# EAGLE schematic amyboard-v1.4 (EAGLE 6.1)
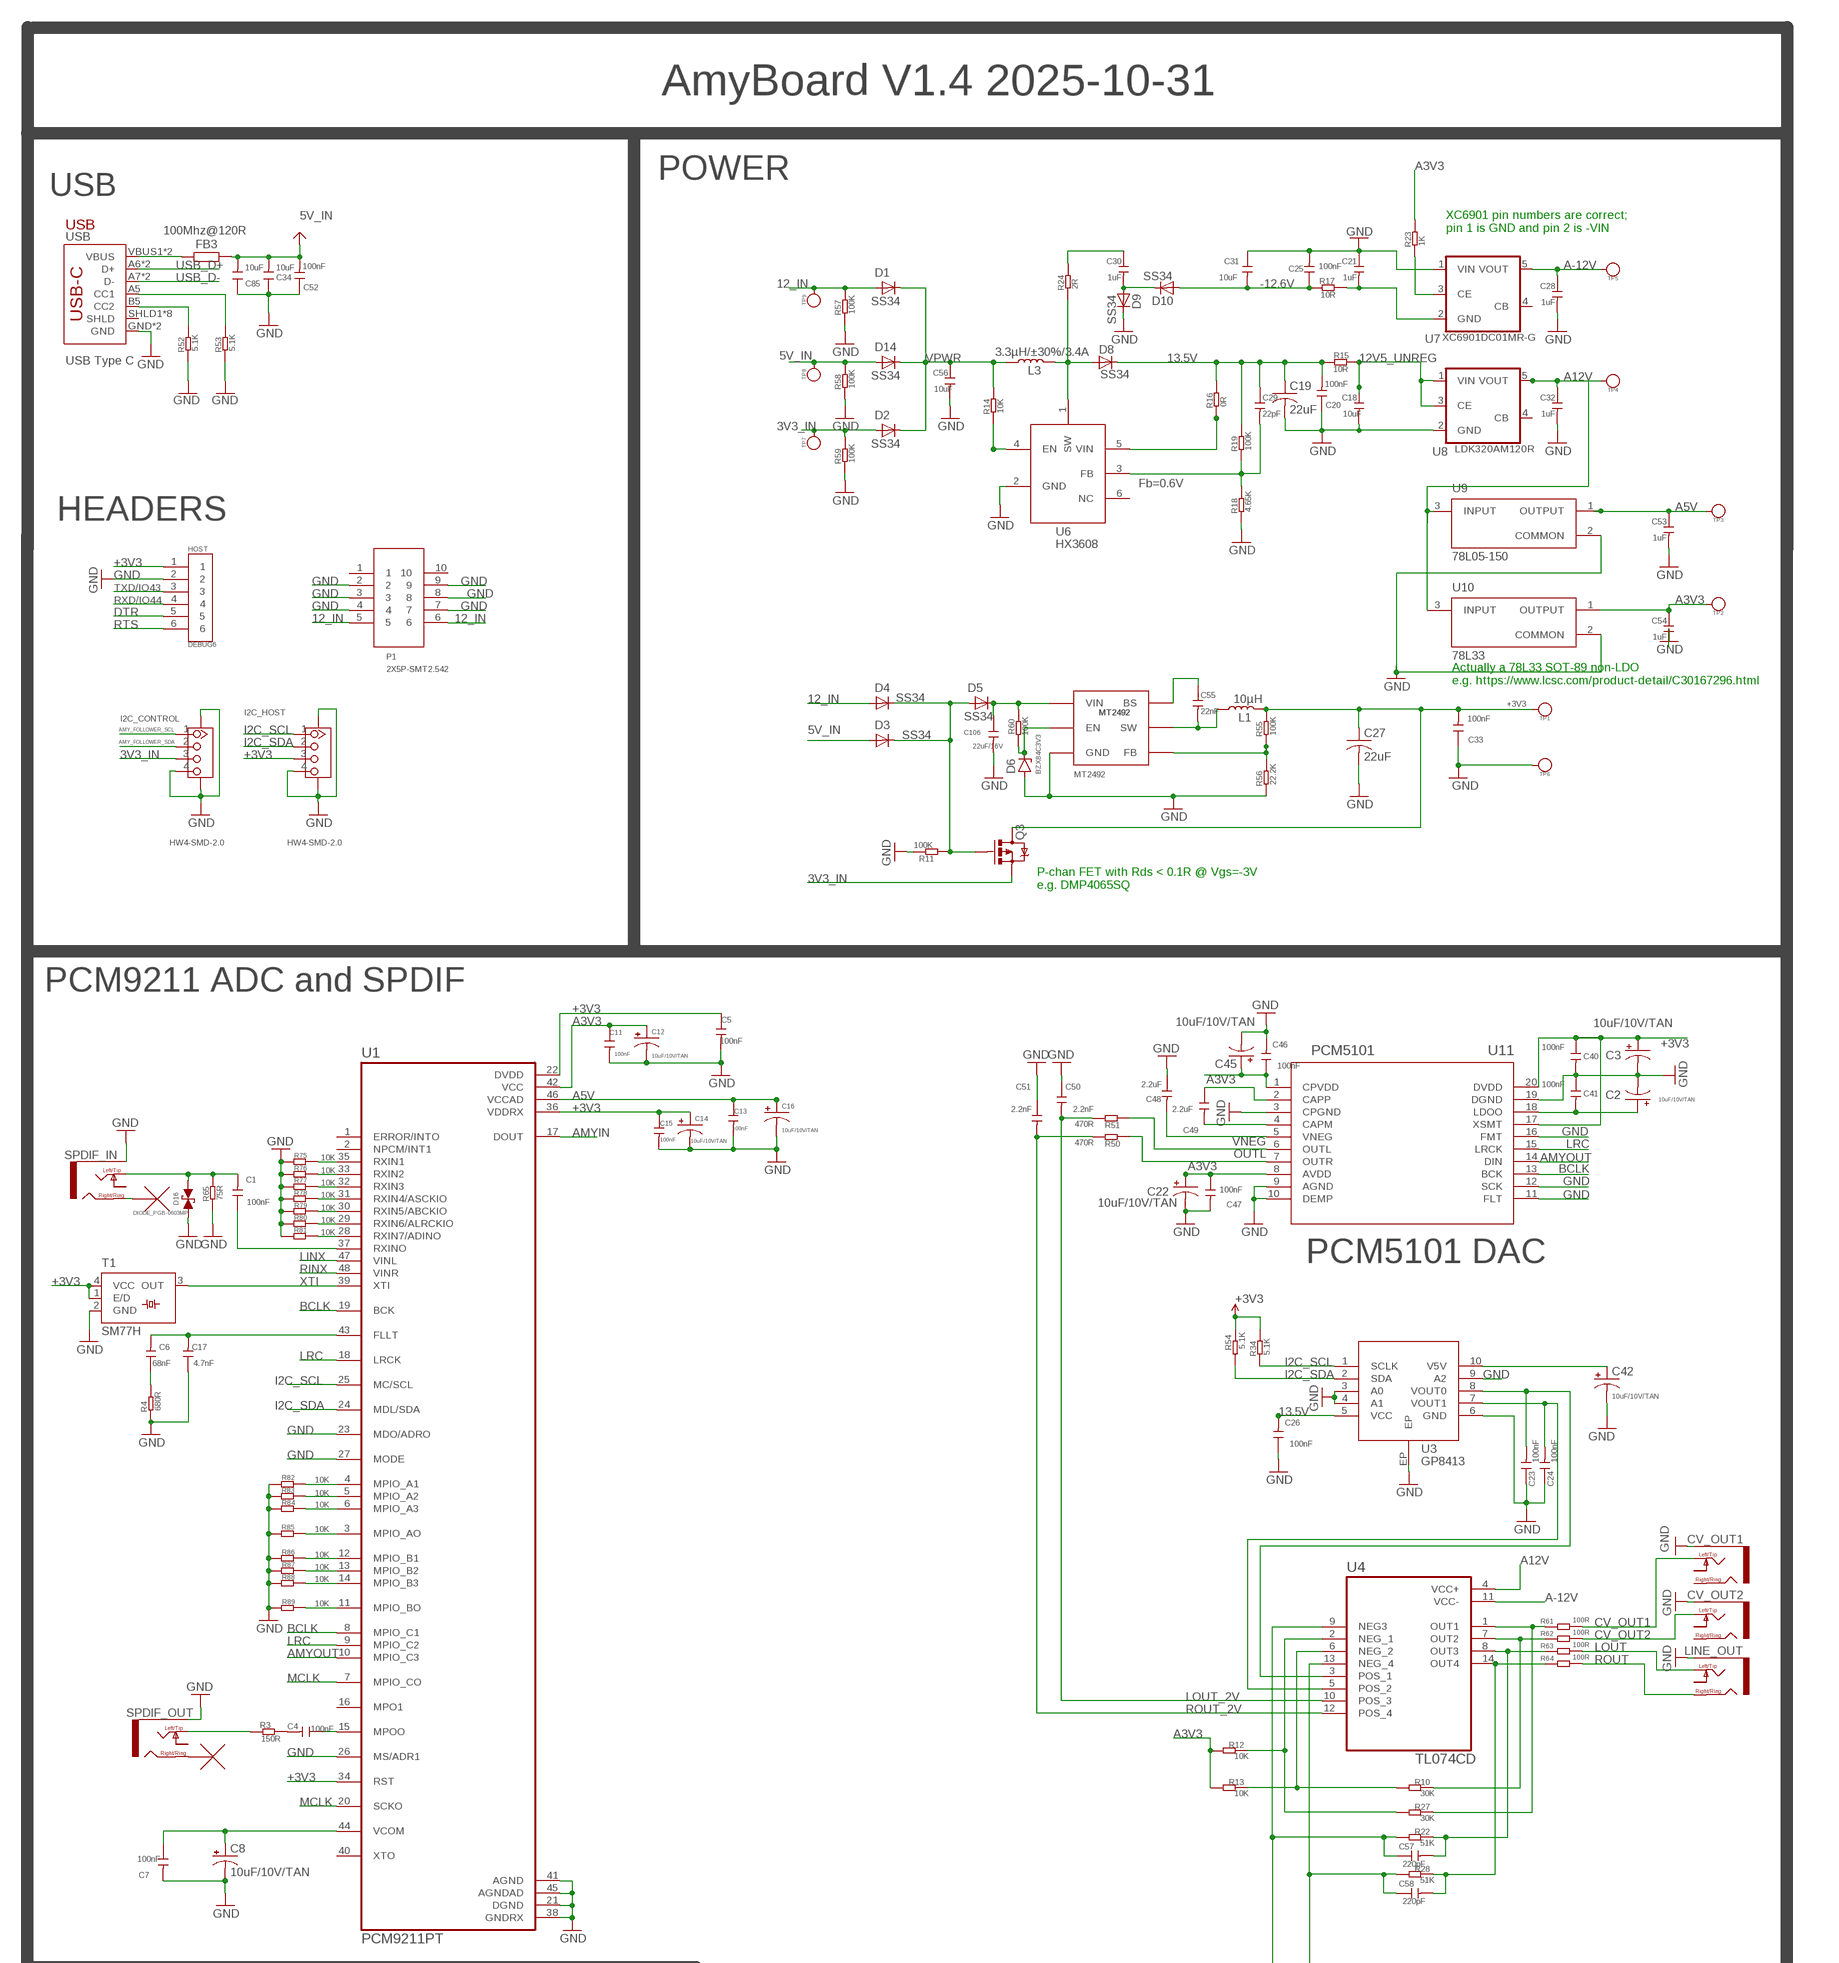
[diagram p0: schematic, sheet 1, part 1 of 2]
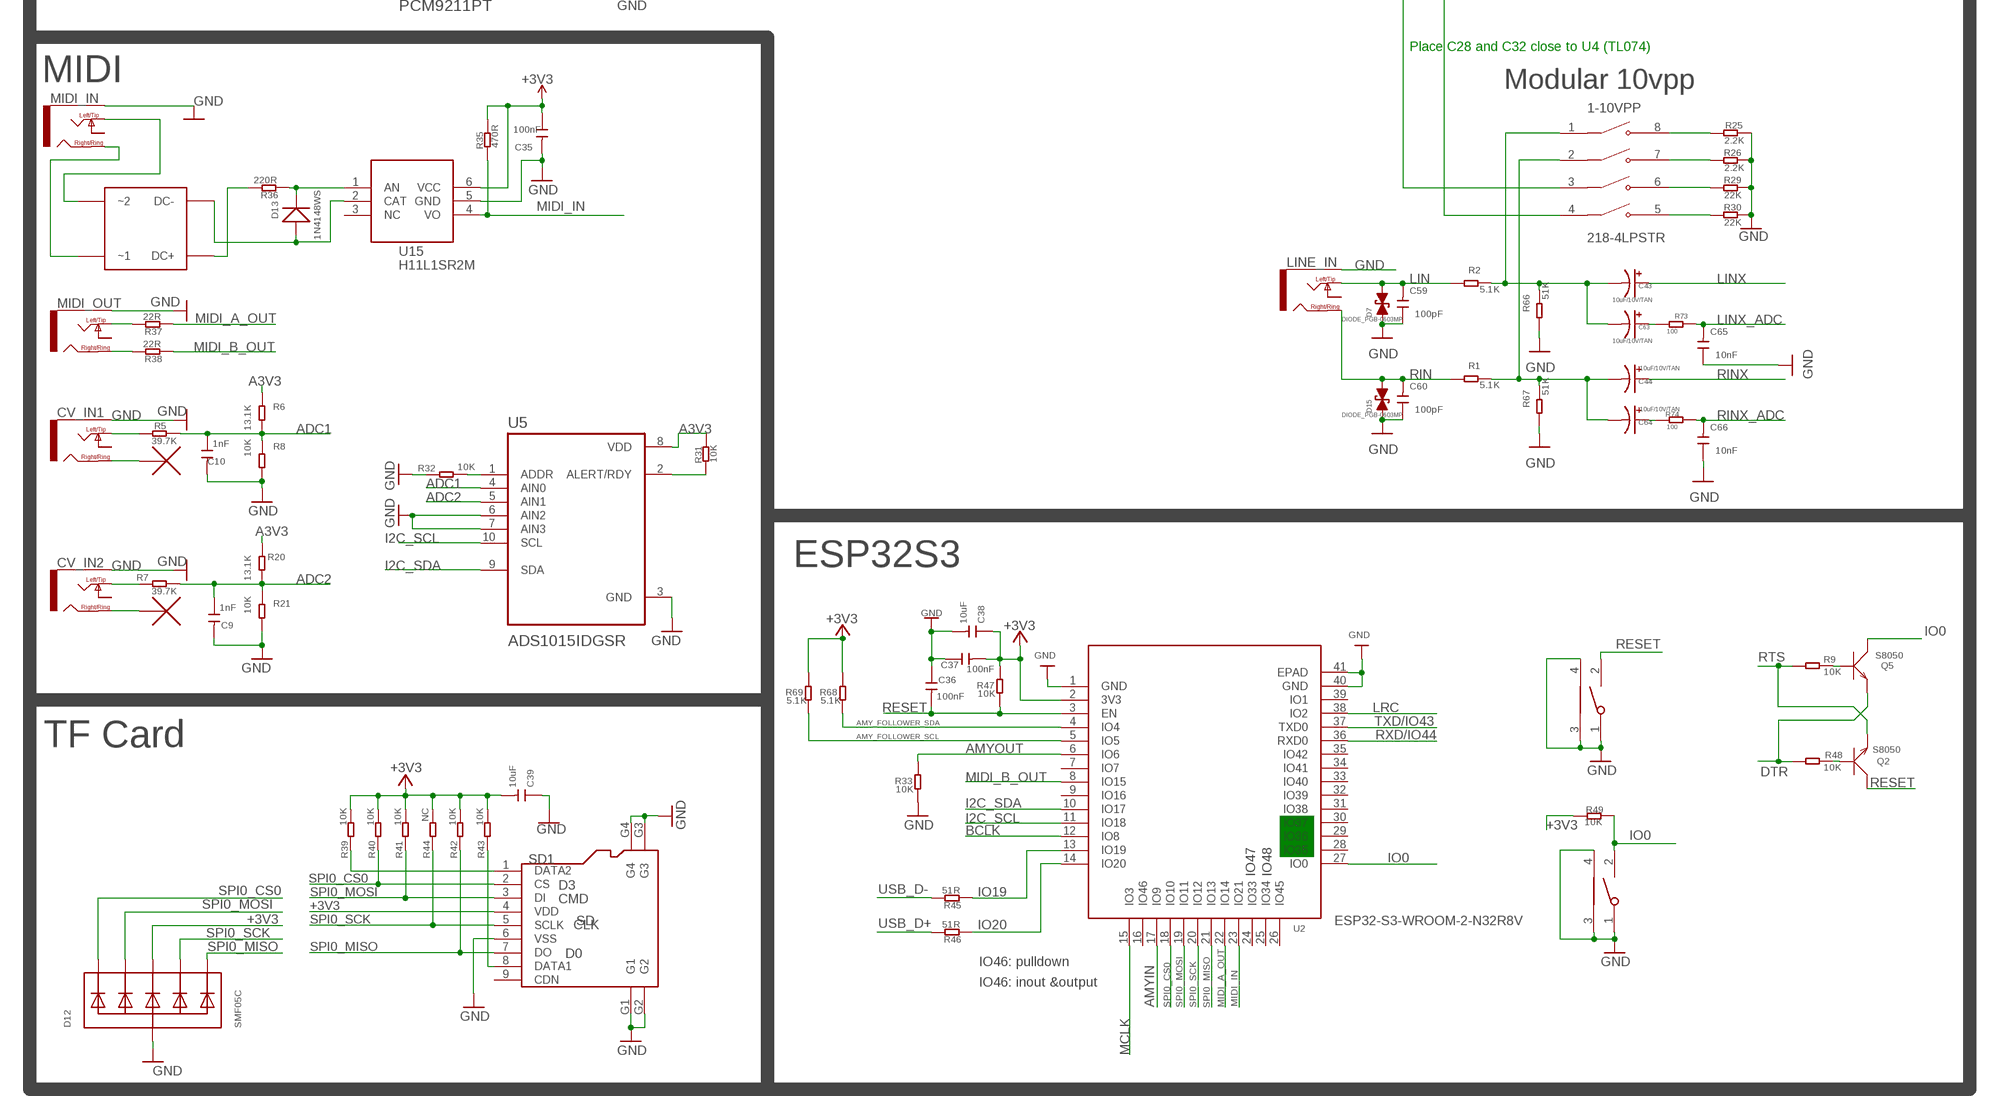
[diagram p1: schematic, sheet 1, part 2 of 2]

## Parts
1-10VPP  218-4LPSTR  [SW_218-4LPSTR]
BOOT  TS24CA  [2*4*3.5MM]
C1  100nF  DISCRETE_C-0402  [DISCRETE_C0402]
C2  10uF/10V/TAN  CPOL-USSMCZ  [SMC_Z]
C3  10uF/10V/TAN  CPOL-USSMCZ  [SMC_Z]
C4  100nF  DISCRETE_C-0402  [DISCRETE_C0402]
C5  100nF  DISCRETE_C-0402  [DISCRETE_C0402]
C6  68nF  DISCRETE_C-0402  [DISCRETE_C0402]
C7  100nF  DISCRETE_C-0402  [DISCRETE_C0402]
C8  10uF/10V/TAN  CPOL-USSMCZ  [SMC_Z]
C9  1nF  DISCRETE_C-0402  [DISCRETE_C0402]
C10  1nF  DISCRETE_C-0402  [DISCRETE_C0402]
C11  100nF  DISCRETE_C-0402  [DISCRETE_C0402]
C12  10uF/10V/TAN  CPOL-USSMCZ  [SMC_Z]
C13  100nF  DISCRETE_C-0402  [DISCRETE_C0402]
C14  10uF/10V/TAN  CPOL-USSMCZ  [SMC_Z]
C15  100nF  DISCRETE_C-0402  [DISCRETE_C0402]
C16  10uF/10V/TAN  CPOL-USSMCZ  [SMC_Z]
C17  4.7nF  DISCRETE_C-0402  [DISCRETE_C0402]
C18  10uF  CAP-0603  [C0603]
C19  22uF  C-USC1206  [C1206]
C20  100nF  DISCRETE_C-0402  [DISCRETE_C0402]
C21  1uF  CAP-0603  [C0603]
C22  10uF/10V/TAN  CPOL-USSMCZ  [SMC_Z]
C23  100nF  DISCRETE_C-0402  [DISCRETE_C0402]
C24  100nF  DISCRETE_C-0402  [DISCRETE_C0402]
C25  100nF  DISCRETE_C-0402  [DISCRETE_C0402]
C26  100nF  DISCRETE_C-0402  [DISCRETE_C0402]
C27  22uF  C-USC1206  [C1206]
C28  1uF  CAP-0603  [C0603]
C29  22pF  CAP-0603  [C0603]
C30  1uF  CAP-0603  [C0603]
C31  10uF  CAP-0603  [C0603]
C32  1uF  CAP-0603  [C0603]
C33  100nF  DISCRETE_C-0402  [DISCRETE_C0402]
C34  10uF  DISCRETE_C-0603  [DISCRETE_C0603]
C35  100nF  DISCRETE_C-0402  [DISCRETE_C0402]
C36  100nF  DISCRETE_C-0402  [DISCRETE_C0402]
C37  100nF  DISCRETE_C-0402  [DISCRETE_C0402]
C38  10uF  DISCRETE_C-0603  [DISCRETE_C0603]
C39  10uF  DISCRETE_C-0603  [DISCRETE_C0603]
C40  100nF  DISCRETE_C-0402  [DISCRETE_C0402]
C41  100nF  DISCRETE_C-0402  [DISCRETE_C0402]
C42  10uF/10V/TAN  CPOL-USSMCZ  [SMC_Z]
C43  10uF/10V/TAN  CPOL-USSMCZ  [SMC_Z]
C44  10uF/10V/TAN  CPOL-USSMCZ  [SMC_Z]
C45  10uF/10V/TAN  CPOL-USSMCZ  [SMC_Z]
C46  100nF  DISCRETE_C-0402  [DISCRETE_C0402]
C47  100nF  DISCRETE_C-0402  [DISCRETE_C0402]
C48  2.2uF  DISCRETE_C-0402  [DISCRETE_C0402]
C49  2.2uF  DISCRETE_C-0402  [DISCRETE_C0402]
C50  2.2nF  DISCRETE_C-0402  [DISCRETE_C0402]
C51  2.2nF  DISCRETE_C-0402  [DISCRETE_C0402]
C52  100nF  DISCRETE_C-0402  [DISCRETE_C0402]
C53  1uF  CAP-0603  [C0603]
C54  1uF  CAP-0603  [C0603]
C55  22nF  CAP-0603  [C0603]
C56  10uF  CAP-0603  [C0603]
C57  220pF  DISCRETE_C-0402  [DISCRETE_C0402]
C58  220pF  DISCRETE_C-0402  [DISCRETE_C0402]
C59  100pF  DISCRETE_C-0402  [DISCRETE_C0402]
C60  100pF  DISCRETE_C-0402  [DISCRETE_C0402]
C63  10uF/10V/TAN  CPOL-USSMCZ  [SMC_Z]
C64  10uF/10V/TAN  CPOL-USSMCZ  [SMC_Z]
C65  10nF  DISCRETE_C-0402  [DISCRETE_C0402]
C66  10nF  DISCRETE_C-0402  [DISCRETE_C0402]
C85  10uF  DISCRETE_C-0603  [DISCRETE_C0603]
C106  22uF/16V  C-0603  [0603]
CV_IN1  NV-PJ3410_STEREO  [NV-PJ3410_SOCKET]
CV_IN2  NV-PJ3410_STEREO  [NV-PJ3410_SOCKET]
CV_OUT1  NV-PJ3410_STEREO  [NV-PJ3410_SOCKET]
CV_OUT2  NV-PJ3410_STEREO  [NV-PJ3410_SOCKET]
D1  SS34  DIODE-DO-214AC  [DO-214AC]
D2  SS34  DIODE-DO-214AC  [DO-214AC]
D3  SS34  DIODE-DO-214AC  [DO-214AC]
D4  SS34  DIODE-DO-214AC  [DO-214AC]
D5  SS34  DIODE-DO-214AC  [DO-214AC]
D6  BZX84C3V3  BZX84CSMD  [TO236]
D7  DIODE_PGB-0603MP  [DIODE_PGB-0603MP]
D8  SS34  DIODE-DO-214AC  [DO-214AC]
D9  SS34  DIODE-DO-214AC  [DO-214AC]
D10  SS34  DIODE-DO-214AC  [DO-214AC]
D12  SMF05C  TVSARRAY_5LANE  [SOT363]
D13  1N4148WS  D'0805'  [SOD323]
D14  SS34  DIODE-DO-214AC  [DO-214AC]
D15  DIODE_PGB-0603MP  [DIODE_PGB-0603MP]
D16  DIODE_PGB-0603MP  [DIODE_PGB-0603MP]
FB3  100Mhz@120R  R-EU_R0805  [R0805]
HOST  DEBUG6  [DEBUG*6]
I2C_CONTROL  HW4-SMD-2.0  GROVE-CONNECTOR-SMD'90D'  [HW4-SMD-2.0-90D]
I2C_HOST  HW4-SMD-2.0  GROVE-CONNECTOR-SMD'90D'  [HW4-SMD-2.0-90D]
L1  10µH  INDUCTOR-CR54-3.3UH  [CR54]
L3  3.3µH/±30%/3.4A  INDUCTOR-CR54-3.3UH  [CR54]
LINE_IN  NV-PJ3410_STEREO  [NV-PJ3410_SOCKET]
LINE_OUT  NV-PJ3410_STEREO  [NV-PJ3410_SOCKET]
MB14F  MB14F  [MBF]
MIDI_IN  NV-PJ3410_STEREO  [NV-PJ3410_SOCKET]
MIDI_OUT  NV-PJ3410_STEREO  [NV-PJ3410_SOCKET]
P1  2X5P-SMT2.542  [2*5P-SMT2.54-HORN]
PCM5101  U11  PCM5101APW  [PW20_TEX]
Q2  S8050  TRANSISTOR-NPN-SOT23  [SOT23]
Q3  DMP4065SQ  MOSFET-PCHANNEL  [SOT23-3]
Q5  S8050  TRANSISTOR-NPN-SOT23  [SOT23]
R1  5.1K  DISCRETE_R-0402  [DISCRETE_R0402]
R2  5.1K  DISCRETE_R-0402  [DISCRETE_R0402]
R3  150R  DISCRETE_R-0402  [DISCRETE_R0402]
R4  680R  DISCRETE_R-0402  [DISCRETE_R0402]
R5  39.7K  DISCRETE_R-0402  [DISCRETE_R0402]
R6  13.1K  DISCRETE_R-0402  [DISCRETE_R0402]
R7  39.7K  DISCRETE_R-0402  [DISCRETE_R0402]
R8  10K  DISCRETE_R-0402  [DISCRETE_R0402]
R9  10K  DISCRETE_R-0402  [DISCRETE_R0402]
R10  30K  DISCRETE_R-0402  [DISCRETE_R0402]
R11  100K  DISCRETE_R-0402  [DISCRETE_R0402]
R12  10K  DISCRETE_R-0402  [DISCRETE_R0402]
R13  10K  DISCRETE_R-0402  [DISCRETE_R0402]
R14  10K  DISCRETE_R-0402  [DISCRETE_R0402]
R15  10R  R-0603  [R0603]
R16  0R  DISCRETE_R-0402  [DISCRETE_R0402]
R17  10R  DISCRETE_R-0402  [DISCRETE_R0402]
R18  4.65K  DISCRETE_R-0402  [DISCRETE_R0402]
R19  100K  DISCRETE_R-0402  [DISCRETE_R0402]
R20  13.1K  DISCRETE_R-0402  [DISCRETE_R0402]
R21  10K  DISCRETE_R-0402  [DISCRETE_R0402]
R22  51K  DISCRETE_R-0402  [DISCRETE_R0402]
R23  1K  DISCRETE_R-0402  [DISCRETE_R0402]
R24  2R  DISCRETE_R-0402  [DISCRETE_R0402]
R25  2.2K  DISCRETE_R-0402  [DISCRETE_R0402]
R26  2.2K  DISCRETE_R-0402  [DISCRETE_R0402]
R27  30K  DISCRETE_R-0402  [DISCRETE_R0402]
R28  51K  DISCRETE_R-0402  [DISCRETE_R0402]
R29  22K  DISCRETE_R-0402  [DISCRETE_R0402]
R30  22K  DISCRETE_R-0402  [DISCRETE_R0402]
R31  10K  DISCRETE_R-0402  [DISCRETE_R0402]
R32  10K  DISCRETE_R-0402  [DISCRETE_R0402]
R33  10K  DISCRETE_R-0402  [DISCRETE_R0402]
R34  5.1K  DISCRETE_R-0402  [DISCRETE_R0402]
R35  470R  DISCRETE_R-0402  [DISCRETE_R0402]
R36  220R  DISCRETE_R-0402  [DISCRETE_R0402]
R37  22R  DISCRETE_R-0402  [DISCRETE_R0402]
R38  22R  DISCRETE_R-0402  [DISCRETE_R0402]
R39  10K  DISCRETE_R-0402  [DISCRETE_R0402]
R40  10K  DISCRETE_R-0402  [DISCRETE_R0402]
R41  10K  DISCRETE_R-0402  [DISCRETE_R0402]
R42  10K  DISCRETE_R-0402  [DISCRETE_R0402]
R43  10K  DISCRETE_R-0402  [DISCRETE_R0402]
R44  NC  DISCRETE_R-0402  [DISCRETE_R0402]
R45  51R  DISCRETE_R-0402  [DISCRETE_R0402]
R46  51R  DISCRETE_R-0402  [DISCRETE_R0402]
R47  10K  DISCRETE_R-0402  [DISCRETE_R0402]
R48  10K  DISCRETE_R-0402  [DISCRETE_R0402]
R49  10K  DISCRETE_R-0402  [DISCRETE_R0402]
R50  470R  DISCRETE_R-0402  [DISCRETE_R0402]
R51  470R  DISCRETE_R-0402  [DISCRETE_R0402]
R52  5.1K  DISCRETE_R-0402  [DISCRETE_R0402]
R53  5.1K  DISCRETE_R-0402  [DISCRETE_R0402]
R54  5.1K  DISCRETE_R-0402  [DISCRETE_R0402]
R55  100K  DISCRETE_R-0402  [DISCRETE_R0402]
R56  22.2K  DISCRETE_R-0402  [DISCRETE_R0402]
R57  100K  DISCRETE_R-0402  [DISCRETE_R0402]
R58  100K  DISCRETE_R-0402  [DISCRETE_R0402]
R59  100K  DISCRETE_R-0402  [DISCRETE_R0402]
R60  100K  DISCRETE_R-0402  [DISCRETE_R0402]
R61  100R  DISCRETE_R-0402  [DISCRETE_R0402]
R62  100R  DISCRETE_R-0402  [DISCRETE_R0402]
R63  100R  DISCRETE_R-0402  [DISCRETE_R0402]
R64  100R  DISCRETE_R-0402  [DISCRETE_R0402]
R65  75R  DISCRETE_R-0402  [DISCRETE_R0402]
R66  51K  DISCRETE_R-0402  [DISCRETE_R0402]
R67  51K  DISCRETE_R-0402  [DISCRETE_R0402]
R68  5.1K  DISCRETE_R-0402  [DISCRETE_R0402]
R69  5.1K  DISCRETE_R-0402  [DISCRETE_R0402]
R73  100  DISCRETE_R-0402  [DISCRETE_R0402]
R74  100  DISCRETE_R-0402  [DISCRETE_R0402]
R75  10K  DISCRETE_R-0402  [DISCRETE_R0402]
R76  10K  DISCRETE_R-0402  [DISCRETE_R0402]
R77  10K  DISCRETE_R-0402  [DISCRETE_R0402]
R78  10K  DISCRETE_R-0402  [DISCRETE_R0402]
R79  10K  DISCRETE_R-0402  [DISCRETE_R0402]
R80  10K  DISCRETE_R-0402  [DISCRETE_R0402]
R81  10K  DISCRETE_R-0402  [DISCRETE_R0402]
R82  10K  DISCRETE_R-0402  [DISCRETE_R0402]
R83  10K  DISCRETE_R-0402  [DISCRETE_R0402]
R84  10K  DISCRETE_R-0402  [DISCRETE_R0402]
R85  10K  DISCRETE_R-0402  [DISCRETE_R0402]
R86  10K  DISCRETE_R-0402  [DISCRETE_R0402]
R87  10K  DISCRETE_R-0402  [DISCRETE_R0402]
R88  10K  DISCRETE_R-0402  [DISCRETE_R0402]
R89  10K  DISCRETE_R-0402  [DISCRETE_R0402]
RST  TS24CA  [2*4*3.5MM]
SD1  SD  HOLDER-MICROSD-9P  [9P-SMD-W/-RING]
SPDIF_IN  NV-PJ3410_STEREO  [NV-PJ3410_SOCKET]
SPDIF_OUT  NV-PJ3410_STEREO  [NV-PJ3410_SOCKET]
T1  SM77H  [SM77H]
TP1  PAD-TEST-POINT-CIRCLE'3535'  [TP_3535]
TP2  PAD-TEST-POINT-CIRCLE'3535'  [TP_3535]
TP3  PAD-TEST-POINT-CIRCLE'3535'  [TP_3535]
TP4  PAD-TEST-POINT-CIRCLE'3535'  [TP_3535]
TP5  PAD-TEST-POINT-CIRCLE'3535'  [TP_3535]
TP6  PAD-TEST-POINT-CIRCLE'3535'  [TP_3535]
TP7  PAD-TEST-POINT-CIRCLE'3535'  [TP_3535]
TP8  PAD-TEST-POINT-CIRCLE'3535'  [TP_3535]
TP9  PAD-TEST-POINT-CIRCLE'3535'  [TP_3535]
U1  PCM9211PT  [QFP50P900X900X160-48N]
U2  ESP32­S2­SOLO  [ESP32-­S2-­SOLO]
U3  GP8413  [ESOP-10-EP-150MIL]
U4  TL074CD  [SOIC127P600X175-14N]
U5  ADS1015IDGSR  [SOP50P490X110-10N]
U6  HX3608  [SOT-23-6]
U7  TS5205  [SOT25]
U8  TS5205  [SOT25]
U9  78L05-150  UA78L05ACPKG4  [VREG_UA78L05ACPKG4]
U10  78L33  UA78L05ACPKG4  [VREG_UA78L05ACPKG4]
U12  MT2492  [SOT23-6]
U15  H11L1SR2M  [SOP-6-2.54MM]
U$1  NC_MARKER  (no package)
U$2  NC_MARKER  (no package)
U$5  NC_MARKER  (no package)
U$6  NC_MARKER  (no package)
USB  USB-C  USB_C5  [USB-C-16P-5]

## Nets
3V3_IN: D2.A I2C_CONTROL.3 Q3.2(S) R59.1 TP7.T
5V_IN: C34.2 C52.2 C85.2 D3.A D14.A FB3.2 R58.1 TP8.T ; supply symbol labelled VBUS
12_IN: D1.A D4.A P1.5 P1.6 R57.1 TP9.T
12V5_UNREG: C18.1 R15.1 U8.1(VIN) U8.3(CE)
13.5V: C19.1 C20.2 C26.2 C29.1 D8.C R15.2 R16.1 R19.1 U3.5(VCC)
+3V3: C3.+ C5.1 C14.+ C15.1 C27.1 C33.2 C35.1 C37.2 C38.1 C39.2 C40.1 D12.4(C3) HOST.1 I2C_HOST.3 L1.P$2 PCM5101.17(XSMT) PCM5101.20(DVDD) Q3.3(D) R34.1 R35.1 R39.2 R40.2 R41.2 R42.2 R43.2 R44.2 R47.2 R49.2 R54.1 R55.1 R68.2 R69.2 SD1.4(VDD) T1.1(E/D) T1.4(VCC) TP1.T U1.22(DVDD) U1.34(RST) U1.36(VDDRX) U2.2(3V3) U15.6(VCC)
-12.6V: C25.1 C31.2 D10.A R17.2
A3V3: C11.1 C12.+ C22.+ C45.+ C46.1 C47.1 C54.1 PCM5101.1(CPVDD) PCM5101.8(AVDD) R6.2 R12.2 R13.2 R20.2 R23.1 R31.1 TP2.T U1.42(VCC) U5.8(VDD) U10.1(OUTPUT)
A5V: C13.1 C16.+ C53.1 TP3.T U1.46(VCCAD) U9.1(OUTPUT)
A12V: C32.1 TP4.T U4.4(VCC+) U8.5(VOUT) U9.3(INPUT) U10.3(INPUT)
A-12V: C28.1 TP5.T U4.11(VCC-) U7.5(VOUT)
ADC1: C10.1 R5.1 R6.1 R8.2 U5.4(AIN0)
ADC2: C9.1 R7.1 R20.1 R21.2 U5.5(AIN1)
AMY_FOLLOWER_SCL: I2C_CONTROL.1 R69.1 U2.5(IO5)
AMY_FOLLOWER_SDA: I2C_CONTROL.2 R68.1 U2.4(IO4)
AMYIN: U1.17(DOUT) U2.17(IO9)
AMYOUT: PCM5101.14(DIN) R33.2 U1.10(MPIO_C3) U2.6(IO6)
BCLK: PCM5101.13(BCK) U1.8(MPIO_C1) U1.19(BCK) U2.12(IO8)
CV_OUT1: CV_OUT1.LEFT/TIP(TIP) R61.1
CV_OUT2: CV_OUT2.LEFT/TIP(TIP) R62.1
DTR: HOST.5 Q5.2(E) R48.2
ENABLE: R14.2 U6.4(EN)
GND: BOOT.1 BOOT.3 BOOT.4 C2.- C3.- C5.2 C7.2 C8.- C9.2 C10.2 C11.2 C12.- C13.2 C14.- C15.2 C16.- C17.1 C18.2 C19.2 C20.1 C21.1 C22.- C23.1 C24.1 C25.2 C26.1 C27.2 C28.2 C31.1 C32.2 C33.1 C34.1 C35.2 C36.1 C37.1 C38.2 C39.1 C40.2 C41.1 C42.- C45.- C46.2 C47.2 C48.1 C50.1 C51.1 C52.1 C53.2 C54.2 C56.2 C59.1 C60.1 C65.1 C66.1 C85.1 C106.2 CV_IN1.GND(EARTH) CV_IN2.GND(EARTH) CV_OUT1.GND(EARTH) CV_OUT2.GND(EARTH) D6.A D7.1 D9.C D12.2(A) D15.1 D16.1 HOST.2 I2C_CONTROL.4 I2C_CONTROL.SS1 I2C_CONTROL.SS2 I2C_HOST.4 I2C_HOST.SS1 I2C_HOST.SS2 LINE_IN.GND(EARTH) LINE_OUT.GND(EARTH) MIDI_IN.GND(EARTH) MIDI_OUT.GND(EARTH) P1.2 P1.3 P1.4 P1.7 P1.8 P1.9 PCM5101.3(CPGND) PCM5101.9(AGND) PCM5101.10(DEMP) PCM5101.11(FLT) PCM5101.12(SCK) PCM5101.16(FMT) PCM5101.19(DGND) R4.2 R8.1 R11.1 R18.2 R21.1 R25.1 R26.1 R29.1 R30.1 R32.1 R33.1 R52.2 R53.2 R56.2 R57.2 R58.2 R59.2 R65.2 R66.2 R67.2 R75.2 R76.2 R77.2 R78.2 R79.2 R80.2 R81.2 R82.2 R83.2 R84.2 R85.2 R86.2 R87.2 R88.2 R89.2 RST.1 RST.3 RST.4 SD1.6(VSS) SD1.G1 SD1.G2 SD1.G3 SD1.G4 SPDIF_IN.GND(EARTH) SPDIF_OUT.GND(EARTH) T1.2(GND) TP6.T U1.21(DGND) U1.23(MDO/ADRO) U1.26(MS/ADR1) U1.27(MODE) U1.38(GNDRX) U1.41(AGND) U1.45(AGNDAD) U2.1(GND) U2.40(GND) U2.41(EPAD) U3.3(A0) U3.4(A1) U3.6(GND) U3.9(A2) U3.EP U5.3(GND) U5.6(AIN2) U5.7(AIN3) U6.2(GND) U7.1(VIN) U8.2(GND) U9.2(COMMON) U10.2(COMMON) U12.2(GND) U15.5(GND) USB.GND USB.GND2(GND)
I2C_SCL: I2C_HOST.1 R34.2 U1.25(MC/SCL) U2.11(IO18) U3.1(SCLK) U5.10(SCL)
I2C_SDA: I2C_HOST.2 R54.2 U1.24(MDL/SDA) U2.10(IO17) U3.2(SDA) U5.9(SDA)
IO0: BOOT.2 Q5.3(C) R49.1 U2.27(IO0)
IO19: R45.2 U2.13(IO19)
IO20: R46.2 U2.14(IO20)
LIN: C59.2 D7.2 LINE_IN.LEFT/TIP(TIP) R2.2
LINX: C43.+ U1.47(VINL)
LINX_ADC: C65.2 R73.1
LOUT: LINE_OUT.LEFT/TIP(TIP) R63.1
LOUT_2V: C50.2 R51.1 U4.10(POS_3)
LRC: PCM5101.15(LRCK) U1.9(MPIO_C2) U1.18(LRCK) U2.38(IO2)
MCLK: U1.7(MPIO_CO) U1.20(SCKO) U2.15(IO3)
MIDI_A_OUT: R37.2 U2.22(IO14)
MIDI_B_OUT: R38.2 U2.8(IO15)
MIDI_IN: R35.2 U2.23(IO21) U15.4(VO)
N$1: C1.1 U1.37(RXINO)
N$2: C4.2 R3.1
N$3: C4.1 U1.15(MPOO)
N$4: 1-10VPP.1 C43.- C63.- R2.1 R66.1
N$5: 1-10VPP.2 C44.- C64.- R1.1 R67.1
N$6: C7.1 C8.+ U1.44(VCOM)
N$7: C6.2 C17.2 U1.43(FLLT)
N$8: C6.1 R4.1
N$9: SPDIF_OUT.RIGHT/RING(RING) U$1.P$1
N$10: SPDIF_IN.RIGHT/RING(RING) U$2.P$1
N$13: CV_IN2.LEFT/TIP(TIP) R7.2
N$14: CV_IN2.RIGHT/RING(RING) U$6.P$1
N$15: C21.2 R17.1 U7.2(GND)
N$16: D13.+ MB14F.DCMINUS(DC-) U15.2(CAT)
N$17: CV_IN1.RIGHT/RING(RING) U$5.P$1
N$18: C23.2 U3.8(VOUT0) U4.3(POS_1)
N$19: CV_IN1.LEFT/TIP(TIP) R5.2
N$20: C24.2 U3.7(VOUT1) U4.5(POS_2)
N$21: D8.A L3.P$2 R24.2 U6.1(SW)
N$22: C42.+ U3.10(V5V)
N$23: D3.C D4.C D5.A Q3.1(G) R11.2
N$24: C106.1 D5.C R60.1 U12.5(VIN)
N$25: C55.2 L1.P$1 U12.6(SW)
N$26: R10.1 R62.2 U4.7(OUT2)
N$27: C30.1 R24.1
N$28: R16.2 U6.5(VIN)
N$29: C30.2 D9.A D10.C
N$30: R23.2 U7.3(CE)
N$31: R10.2 R13.1 U4.6(NEG_2)
N$32: R27.1 R61.2 U4.1(OUT1)
N$33: R12.1 R27.2 U4.2(NEG_1)
N$34: Q2.1(B) R48.1
N$35: 1-10VPP.5 R30.2
N$36: 1-10VPP.6 R29.2
N$37: Q5.1(B) R9.1
N$38: R53.1 USB.A5(CC1)
N$39: R52.1 USB.B5(CC2)
N$40: 1-10VPP.8 R25.2
N$41: 1-10VPP.7 R26.2
N$42: FB3.1 USB.VBUS1(VBUS) USB.VBUS2(VBUS)
N$43: R31.2 U5.2(ALERT/RDY)
N$44: 1-10VPP.3 C57.1 R22.2 U4.9(NEG3)
N$45: 1-10VPP.4 C58.1 R28.2 U4.13(NEG_4)
N$46: R32.2 U5.1(ADDR)
N$47: R55.2 R56.1 U12.3(FB)
N$48: C2.+ C41.2 PCM5101.18(LDOO)
N$49: MB14F.DCPLUS(DC+) R36.1
N$50: PCM5101.7(OUTR) R50.2
N$51: C49.2 PCM5101.4(CAPM)
N$52: C49.1 PCM5101.2(CAPP)
N$53: C55.1 U12.1(BS)
N$54: MB14F.AC1(~1) MIDI_IN.RIGHT/RING(RING)
N$55: MB14F.AC2(~2) MIDI_IN.LEFT/TIP(TIP)
N$56: D6.C R60.2 U12.4(EN)
N$57: D13.- R36.2 U15.1(AN)
N$58: MIDI_OUT.LEFT/TIP(TIP) R37.1
N$59: MIDI_OUT.RIGHT/RING(RING) R38.1
N$60: C29.2 R18.1 R19.2 U6.3(FB)
N$61: C58.2 R28.1 R64.2 U4.14(OUT4)
N$63: C57.2 R22.1 R63.2 U4.8(OUT3)
N$67: R75.1 U1.35(RXIN1)
N$68: R76.1 U1.33(RXIN2)
N$69: C63.+ R73.2
N$70: C64.+ R74.2
N$75: R39.1 SD1.1(DATA2)
N$76: R77.1 U1.32(RXIN3)
N$77: R43.1 SD1.8(DATA1)
N$78: R78.1 U1.31(RXIN4/ASCKIO)
N$79: R79.1 U1.30(RXIN5/ABCKIO)
N$80: R80.1 U1.29(RXIN6/ALRCKIO)
N$81: R81.1 U1.28(RXIN7/ADINO)
N$82: R82.1 U1.4(MPIO_A1)
N$83: R83.1 U1.5(MPIO_A2)
N$84: R84.1 U1.6(MPIO_A3)
N$85: R85.1 U1.3(MPIO_AO)
N$86: R86.1 U1.12(MPIO_B1)
N$87: R87.1 U1.13(MPIO_B2)
N$88: R88.1 U1.14(MPIO_B3)
N$89: R89.1 U1.11(MPIO_BO)
OUTL: PCM5101.6(OUTL) R51.2
RESET: C36.2 Q2.3(C) R47.1 RST.2 U2.3(EN)
RIN: C60.2 D15.2 LINE_IN.RIGHT/RING(RING) R1.2
RINX: C44.+ U1.48(VINR)
RINX_ADC: C66.2 R74.1
ROUT: LINE_OUT.RIGHT/RING(RING) R64.1
ROUT_2V: C51.2 R50.1 U4.12(POS_4)
RTS: HOST.6 Q2.2(E) R9.2
RXD/IO44: HOST.4 U2.36(RXD0)
SPDIFIN_SIGNAL: C1.2 D16.2 R65.1 SPDIF_IN.LEFT/TIP(TIP)
SPDIFOUT_SIGNAL: R3.2 SPDIF_OUT.LEFT/TIP(TIP)
SPI0_CS0: D12.1(C1) R40.1 SD1.2(CS) U2.18(IO10)
SPI0_MISO: D12.6(C5) R42.1 SD1.7(DO) U2.21(IO13)
SPI0_MOSI: D12.3(C2) R41.1 SD1.3(DI) U2.19(IO11)
SPI0_SCK: D12.5(C4) R44.1 SD1.5(SCLK) U2.20(IO12)
TXD/IO43: HOST.3 U2.37(TXD0)
USB_D+: R46.1 USB.A6(D+) USB.B6(D+)
USB_D-: R45.1 USB.A7(D-) USB.B7(D-)
VNEG: C48.2 PCM5101.5(VNEG)
VPWR: C56.1 D1.C D2.C D14.C L3.P$1 R14.1
XTI: T1.3(OUT) U1.39(XTI)
Unconnected: CV_IN1.SWITCH(TIP-NORM) CV_IN2.SWITCH(TIP-NORM) CV_OUT1.RIGHT/RING(RING) CV_OUT1.SWITCH(TIP-NORM) CV_OUT2.RIGHT/RING(RING) CV_OUT2.SWITCH(TIP-NORM) LINE_IN.SWITCH(TIP-NORM) LINE_OUT.SWITCH(TIP-NORM) MIDI_IN.SWITCH(TIP-NORM) MIDI_OUT.SWITCH(TIP-NORM) P1.1 P1.10 SD1.9(CDN) SPDIF_IN.SWITCH(TIP-NORM) SPDIF_OUT.SWITCH(TIP-NORM) U1.1(ERROR/INTO) U1.2(NPCM/INT1) U1.16(MPO1) U1.40(XTO) U2.7(IO7) U2.9(IO16) U2.16(IO46) U2.24(IO33) U2.25(IO34) U2.26(IO45) U2.28(IO35) U2.29(IO36) U2.30(IO37) U2.31(IO38) U2.32(IO39) U2.33(IO40) U2.34(IO41) U2.35(IO42) U2.39(IO1) U6.6(NC) U7.4(CB) U8.4(CB) U15.3(NC) USB.SHLD1(SHLD) USB.SHLD2(SHLD) USB.SHLD3(SHLD) USB.SHLD4(SHLD) USB.SHLD5(SHLD) USB.SHLD6(SHLD) USB.SHLD7(SHLD) USB.SHLD8(SHLD)

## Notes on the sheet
- AmyBoard V1.4 2025-10-31
- POWER
- USB
- USB
- XC6901 pin numbers are correct; 
  pin 1 is GND and pin 2 is -VIN
- XC6901DC01MR-G
- USB Type C
- LDK320AM120R
- Fb=0.6V
- HEADERS
- Actually a 78L33 SOT-89 non-LDO 
  e.g. https://www.lcsc.com/product-detail/C30167296.html
- P-chan FET with Rds < 0.1R @ Vgs=-3V
  e.g. DMP4065SQ
- PCM9211 ADC and SPDIF
- PCM5101 DAC
- Place C28 and C32 close to U4 (TL074)
- MIDI | Modular 10vpp
- ESP32S3
- TF Card
- IO47 | IO48
- D3
- CMD
- ESP32-S3-WROOM-2-N32R8V
- CLK
- D0
- IO46: pulldown
- IO46: inout &output

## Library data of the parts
1-10VPP = 218-4LPSTR:218-4LPSTR: Check availability; AVAILABILITY: In Stock; CHECK_PRICES: https://www.snapeda.com/parts/218-4LPSTR/CTS+Components/view-part/?ref=eda; DESCRIPTION: Dip Switch SPST 4 Position Surface Mount Slide (Standard) Actuator 25mA 24VDC; MF: CTS Electrocomponents; MP: 218-4LPSTR; PACKAGE: None; PRICE: None; SNAPEDA_LINK: https://www.snapeda.com/parts/218-4LPSTR/CTS+Components/view-part/?ref=snap
BOOT RST = sale:TS24CA
C1 C4-C7 C9-C11 C13 C15 C17 C20 C23-C26 C33-C41 C46-C52 C57-C60 C65 C66 C85 = A9G:DISCRETE_C*: Ceramic Capacitors
C2 C3 C8 C12 C14 C16 C22 C42-C45 C63 C64 = rcl:CPOL-US: POLARIZED CAPACITOR, American symbol
C18 C21 C28-C32 C53-C56 = Discrete-new:CAP: Ceramic Capacitors
C19 C27 = adafruit:C-US: CAPACITOR, American symbol
C106 = Discrete:C*: Ceramic Capacitors
CV_IN1 CV_IN2 CV_OUT1 CV_OUT2 LINE_IN LINE_OUT MIDI_IN MIDI_OUT SPDIF_IN SPDIF_OUT = PJ3410_sockets:NV-PJ3410_STEREO: PJ3410 socket stereo with switch
D1-D5 D8-D10 D14 = diode:DIODE-: DIODE
D6 = diode@1:BZX84CSMD: Z DIODE
D7 D15 D16 = 52101-101-REV-A_v16:DIODE_PGB-0603: ESD SUPPRESSOR
D12 = microbuilder:TVSARRAY_5LANE: Voltage Transient Suppressor Array SOT363 SMF05C - 100W 5V: Digikey - SMF05CT1GOSCT-ND
D13 = Discrete:D*
FB3 = rcl:R-EU_: RESISTOR, European symbol
HOST = Makerfabs-Peter:DEBUG*6
I2C_CONTROL I2C_HOST = Connector-new:GROVE-CONNECTOR-SMD: 4P-SMD-2.0:320110030;4P-SMD-2.0-90D:320110032
L1 = SparkFun-Coils:INDUCTOR: Inductors; PROD_ID: NDUC-11157; VALUE: 3.3µH/±30%/3.4A
L3 = SparkFun-Coils:INDUCTOR: Inductors; PROD_ID: NDUC-11157
MB14F = dpwe:MB14F: MB14F Bridge Rectifier 1A 40V https://www.lcsc.com/datasheet/lcsc_datasheet_2410121530_GOODWORK-MB14F_C2943867.pdf
P1 = sale:2X5P-SMT2.54
PCM5101 = pcm5101apw:PCM5101APW; COPYRIGHT: Copyright (C) 2022 Ultra Librarian. All rights reserved.; DIGI-KEY_PART_NUMBER_1: PCM5101APW-ND; MANUFACTURER_PART_NUMBER: PCM5101APW; MFR_NAME: Texas Instruments
Q2 Q5 = Discrete:TRANSISTOR-NPN*: NPN audion
Q3 = User-Submitted:MOSFET-PCHANNEL: Generic PMOSFET IRLML2244 - TRANS-11153 (SOT-23 -20V -4.3A) (1.Gate 2.Source 3.Drain) FQP27P06 - COM-10349 (TO-220 -60V -27A) (1.Gate 2.Source 3.Drain); PROD_ID: TRANS-08285
R1-R14 R16-R69 R73-R89 = A9G:DISCRETE_R*
R15 = Discrete:R*
SD1 = Connector:HOLDER-MICROSD-9P
T1 = crystal:SM77H: 3.3V CMOS Clock Oscillator Source: www.pletronics.com .. sm77h%203.3v.pdf; OC_FARNELL: unknown; OC_NEWARK: unknown
TP1-TP9 = Discrete:PAD-TEST-POINT-CIRCLE; PARTNO: DNP
U1 = PCM9211PT:PCM9211PT: Check availability; AVAILABILITY: In Stock; CHECK_PRICES: https://www.snapeda.com/parts/PCM9211PT/Texas+Instruments/view-part/?ref=eda; DESCRIPTION: 216kHz Digital Audio Interface Transceiver (DIX) with Stereo ADC and Routing; MF: Texas Instruments; MP: PCM9211PT; PACKAGE: LQFP-48 Texas Instruments; PRICE: None; SNAPEDA_LINK: https://www.snapeda.com/parts/PCM9211PT/Texas+Instruments/view-part/?ref=snap
U2 = self:ESP32­S2­SOLO
U3 = sale:GP8413
U4 = TL074CD:TL074CD: Check availability; AVAILABILITY: In Stock; CHECK_PRICES: https://www.snapeda.com/parts/TL074CD/Texas+Instruments/view-part/?ref=eda; DESCRIPTION: Quad, 30-V, 3-MHz, high slew rate (13-V/µs), In to V+, JFET-input op amp; MF: Texas Instruments; MP: TL074CD; PACKAGE: SOIC-14 Texas Instruments; PRICE: None; SNAPEDA_LINK: https://www.snapeda.com/parts/TL074CD/Texas+Instruments/view-part/?ref=snap
U5 = ADS1015IDGSR:ADS1015IDGSR: Check availability; AVAILABILITY: In Stock; CHECK_PRICES: https://www.snapeda.com/parts/ADS1015IDGSR/Texas+Instruments/view-part/?ref=eda; DESCRIPTION: 12-bit, 3.3-kSPS, 4-channel, delta-sigma ADC with PGA, oscillator, VREF, comparator and I2C; MF: Texas Instruments; MP: ADS1015IDGSR; PACKAGE: VSSOP-10 Texas Instruments; PRICE: None; SNAPEDA_LINK: https://www.snapeda.com/parts/ADS1015IDGSR/Texas+Instruments/view-part/?ref=snap
U6 = self:HX3608
U7 U8 = v-reg:TS5205: 150mA Low Noise LDO Voltage Regulator with Enable TSC [Taiwan Semiconductor Company, Ltd] Source: http://www.taiwansemi.com .. 5205_0409c.pdf
U9 U10 = UA78L05ACPKG4:UA78L05ACPKG4: Check availability; AVAILABILITY: Not in stock; CHECK_PRICES: https://www.snapeda.com/parts/UA78L05ACPKG4/Texas+Instruments/view-part/?ref=eda; DESCRIPTION: V REG 0.1A +5.0V, 78L05, SOT-89-3; Voltage Regulator Type: Fixed; Voltage, Input Max: 20V; Voltage, Output Max: 5V; O...; MF: Texas Instruments; MP: UA78L05ACPKG4; PACKAGE: SOT-89-3 Texas Instruments; PRICE: None; SNAPEDA_LINK: https://www.snapeda.com/parts/UA78L05ACPKG4/Texas+Instruments/view-part/?ref=snap
U12 = dpwe:MT2492: MT2492 600KHz, 16V，2A Synchronous Step-Down Converter https://www.lcsc.com/datasheet/lcsc_datasheet_2408140941_XI-AN-Aerosemi-Tech-MT2492_C89358.pdf
U15 = sale:H11L1SR2M
U$1 U$2 U$5 U$6 = NC_MARKER:NC_MARKER
USB = USBC:USB_C: USB Type C 16Pin Connector Super Speed pins not available on the 16-pin purely SMD connector so this part is best for USB 2.0 implementations. D1 and D2 are tied together enabling D+/- no matter which way the cable is plugged into the connector. The two channel configuration pins (CC1/2) are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

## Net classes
0 default: width 0.203 mm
